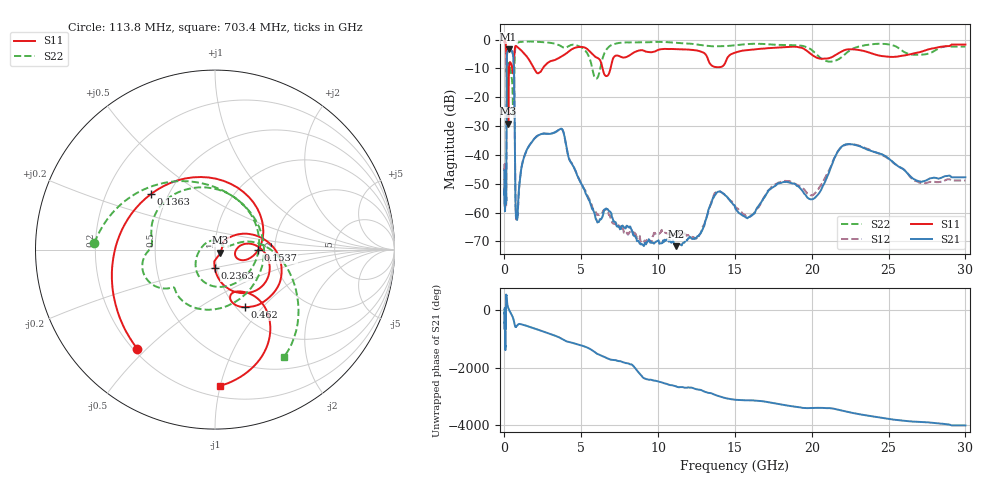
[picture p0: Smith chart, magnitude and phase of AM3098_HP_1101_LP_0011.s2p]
! Date/Time: Thu, Feb 28, 2019 8:45 AM
! Network Analyzer: Agilent Technologies E8364B Rev: A.07.50.67
! Sweep from 0.010 to 30.000 GHz, 1601 Points, Sweep Type: LOG
! Power Supply: 5.022 V, 0.002 A
# Hz S DB R 50
!freq MagS11 AngS11 MagS21 AngS21 MagS12 AngS12 MagS22 AngS22
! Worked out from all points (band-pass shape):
!   1601 points, 10 MHz to 30 GHz, reference 50 ohm
!   highest |S21| = -3.40 dB at 266.5 MHz (marker M1); lowest = -71.7 dB at 11.19 GHz (marker M2)
!   |S21| within 3 dB of the highest: 158.7 MHz to 581.2 MHz (422.6 MHz wide, 114 % of centre)
!   lowest |S11| = -29.2 dB at 249.7 MHz (marker M3), VSWR 1.07, Z = 53.1 - j1.74 ohm
!   |S11| at or under -10 dB: 206.6 MHz to 305.2 MHz (98.65 MHz wide, 38.5 % of centre); 1.92 GHz to 2.494 GHz (573.5 MHz wide, 26 % of centre); 6.38 GHz to 6.903 GHz (522.5 MHz wide, 7.87 % of centre)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
!   |S22| runs from -26.7 to -0.5 dB; largest |S21 - S12| = 0.012
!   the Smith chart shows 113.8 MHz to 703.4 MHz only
!   S11 on the Smith chart (normalised r, x): 113.8 MHz: 0.22, -0.47; 136.3 MHz: 0.40, +0.32; 153.7 MHz: 1.63, -0.01; 236.3 MHz: 0.98, -0.20; 462 MHz: 1.09, -0.81; 703.4 MHz: 0.28, -1.00
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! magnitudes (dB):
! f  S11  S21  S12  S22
! 10 MHz  -0.4  -45.3  -43.7  -0.5
! 38.04 MHz  -0.3  -57.7  -55.2  -0.7
! 113.8 MHz  -3.1  -55.0  -54.7  -3.4
! 136.3 MHz  -6.5  -25.8  -26.0  -10.7
! 144.7 MHz  -8.7  -14.3  -14.2  -10.4
! 153.7 MHz  -12.4  -7.9  -7.9  -9.4
! 236.3 MHz  -19.7  -3.5  -3.5  -8.8
! 249.7 MHz  -29.2  -3.5  -3.4  -9.0
! 266.5 MHz  -18.9  -3.4  -3.3  -9.0
! 462 MHz  -8.8  -3.8  -3.8  -13.0
! 550.5 MHz  -11.7  -5.1  -5.1  -24.6
! 630.1 MHz  -6.2  -12.9  -12.8  -13.6
! 703.4 MHz  -2.4  -50.5  -50.6  -2.9
! 821.5 MHz  -2.5  -62.6  -61.4  -1.3
! 2.084 GHz  -11.4  -33.7  -33.6  -0.7
! 3.723 GHz  -5.8  -31.0  -31.0  -2.4
! 5.959 GHz  -6.1  -62.4  -59.9  -13.6
! 7.926 GHz  -6.1  -64.8  -67.4  -1.0
! 11.19 GHz  -3.3  -71.7  -67.0  -1.1
! 20.1 GHz  -5.6  -55.3  -53.8  -4.1
! 22.56 GHz  -3.4  -36.3  -36.3  -3.5
! 30 GHz  -1.7  -47.8  -48.9  -2.4
